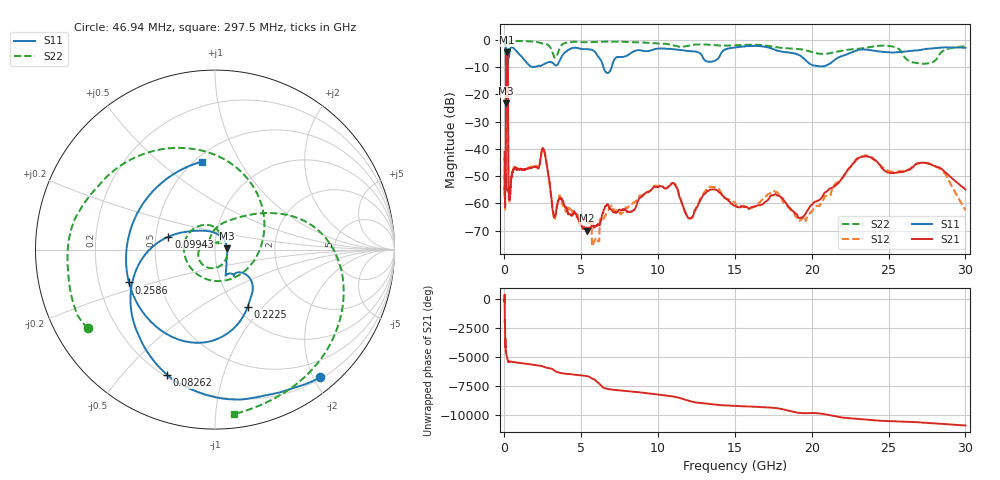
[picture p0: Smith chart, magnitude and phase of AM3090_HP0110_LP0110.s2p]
! Date/Time: Thu, Feb 28, 2019 1:59 PM
! Network Analyzer: Agilent Technologies E8364B Rev: A.07.50.67
! Sweep from 0.010 to 30.000 GHz, 1601 Points, Sweep Type: LOG
! Power Supply: 5.023 V, 0.002 A
# Hz S DB R 50
!freq MagS11 AngS11 MagS21 AngS21 MagS12 AngS12 MagS22 AngS22
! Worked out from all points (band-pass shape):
!   1601 points, 10 MHz to 30 GHz, reference 50 ohm
!   highest |S21| = -4.53 dB at 156 MHz (marker M1); lowest = -70.1 dB at 5.392 GHz (marker M2)
!   |S21| within 3 dB of the highest: 110.7 MHz to 211.5 MHz (100.8 MHz wide, 62.6 % of centre)
!   lowest |S11| = -23.3 dB at 107.7 MHz (marker M3), VSWR 1.15, Z = 57.3 + j0.92 ohm
!   |S11| at or under -10 dB: 98.53 MHz to 213.8 MHz (115.3 MHz wide, 73.8 % of centre); 6.448 GHz to 6.976 GHz (528.6 MHz wide, 7.87 % of centre)
!   |S22| runs from -30.7 to -0.2 dB; largest |S21 - S12| = 0.011
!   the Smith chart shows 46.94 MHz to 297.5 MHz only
!   S11 on the Smith chart (normalised r, x): 46.94 MHz: 0.23, -2.11; 82.62 MHz: 0.21, -0.67; 99.43 MHz: 0.58, +0.09; 222.5 MHz: 1.13, -0.83; 258.6 MHz: 0.33, -0.16; 297.5 MHz: 0.54, +0.70
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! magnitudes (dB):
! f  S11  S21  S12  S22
! 10 MHz  -0.3  -41.1  -44.3  -0.6
! 38.04 MHz  -0.5  -59.4  -59.9  -1.4
! 46.94 MHz  -0.7  -50.9  -49.2  -1.6
! 82.62 MHz  -2.5  -53.6  -50.1  -5.1
! 99.43 MHz  -11.4  -16.7  -16.7  -15.3
! 107.7 MHz  -23.3  -8.6  -8.6  -15.5
! 144.7 MHz  -16.3  -4.6  -4.6  -25.7
! 156 MHz  -15.9  -4.5  -4.5  -21.8
! 222.5 MHz  -8.7  -11.2  -11.2  -11.9
! 258.6 MHz  -5.8  -51.9  -51.7  -1.6
! 297.5 MHz  -6.1  -55.8  -57.8  -0.7
! 550.5 MHz  -2.8  -48.2  -48.0  -0.3
! 2.084 GHz  -9.7  -46.7  -46.3  -0.7
! 2.545 GHz  -9.0  -40.0  -39.8  -1.3
! 3.22 GHz  -8.8  -65.2  -64.3  -6.0
! 5.392 GHz  -3.4  -70.1  -67.1  -0.8
! 5.929 GHz  -4.6  -68.5  -73.0  -0.7
! 7.926 GHz  -5.9  -62.7  -61.3  -0.7
! 10.76 GHz  -3.3  -53.5  -53.2  -1.6
! 19.41 GHz  -6.4  -65.2  -65.2  -3.5
! 23.48 GHz  -3.5  -42.8  -42.4  -2.9
! 30 GHz  -2.9  -54.9  -62.5  -2.3
